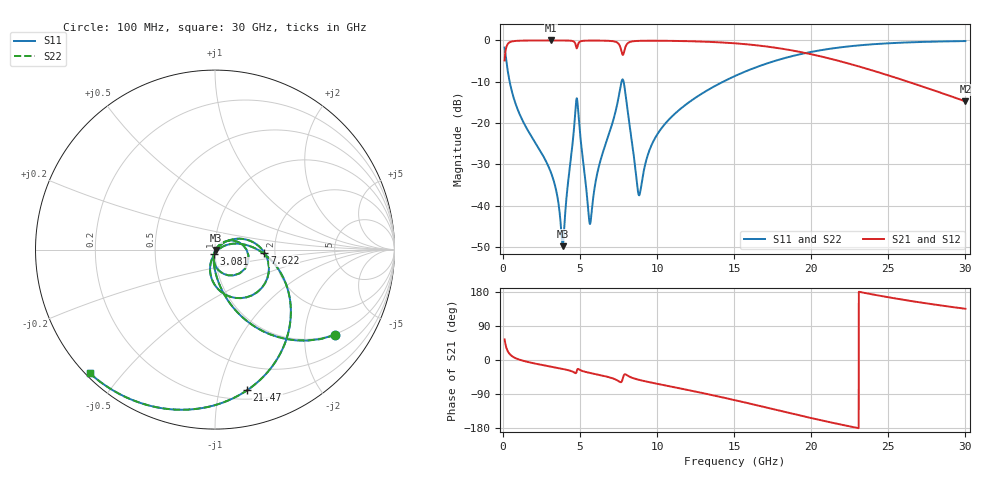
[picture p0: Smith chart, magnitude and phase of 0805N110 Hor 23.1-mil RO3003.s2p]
# GHz S MA R 50
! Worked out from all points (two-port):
!   3201 points, 100 MHz to 30 GHz, reference 50 ohm
!   highest |S21| = -0.02 dB at 3.09 GHz (marker M1); lowest = -14.8 dB at 30 GHz (marker M2)
!   |S21| within 3 dB of the highest: 143.3 MHz to 7.71 GHz (7.567 GHz wide, 193 % of centre); 7.835 GHz to 19.57 GHz (11.73 GHz wide, 85.6 % of centre)
!   lowest |S11| = -49.8 dB at 3.875 GHz (marker M3), VSWR 1.01, Z = 50.3 - j0.137 ohm
!   |S11| at or under -10 dB: 427.9 MHz to 7.687 GHz (7.259 GHz wide, 179 % of centre); 7.822 GHz to 14.28 GHz (6.463 GHz wide, 58.5 % of centre)
!   |S22| runs from -49.8 to -0.2 dB; largest |S21 - S12| = 0
!   S11 on the Smith chart (normalised r, x): 100 MHz: 0.97, -2.83; 3.081 GHz: 0.99, -0.05; 7.622 GHz: 1.76, -0.07; 21.47 GHz: 0.27, -1.22; 30 GHz: 0.01, -0.41
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0.1  0.8201 -35.5  0.5717 54.5  0.5717 54.5  0.8201 -35.5
0.3429375  0.3847 -69.4  0.9224 20.5  0.9224 20.5  0.3847 -69.4
0.62325  0.2218 -80.8  0.9742 9.0  0.9742 9.0  0.2218 -80.8
3.080656  0.02584 -102.7  0.9975 -17.4  0.9975 -17.4  0.02584 -102.7
3.09  0.02557 -102.7  0.9975 -17.5  0.9975 -17.5  0.02557 -102.7
3.874875  0.003219 -25.0  0.9966 -23.7  0.9966 -23.7  0.003219 -25.0
4.725156  0.1676 4.4  0.8643 -34.8  0.8643 -34.8  0.1676 4.4
4.865312  0.1456 -69.5  0.8931 -23.6  0.8931 -23.6  0.1456 -69.5
5.089563  0.05042 -97.9  0.9812 -28.2  0.9812 -28.2  0.05042 -97.9
5.528719  0.008627 -74.7  0.9933 -33.2  0.9933 -33.2  0.008627 -74.7
5.668875  0.006206 -15.3  0.9939 -34.4  0.9939 -34.4  0.006206 -15.3
6.182781  0.028 39.3  0.9937 -38.9  0.9937 -38.9  0.028 39.3
7.621719  0.2763 -3.7  0.8148 -58.6  0.8148 -58.6  0.2763 -3.7
7.892688  0.2634 -75.5  0.7782 -37.8  0.7782 -37.8  0.2634 -75.5
8.817719  0.0133 -46.0  0.9865 -52.3  0.9865 -52.3  0.0133 -46.0
9.434406  0.04327 20.5  0.9902 -58.0  0.9902 -58.0  0.04327 20.5
10.06978  0.07584 21.2  0.9896 -63.4  0.9896 -63.4  0.07584 21.2
15.05  0.3703 -17.2  0.9209 -106.1  0.9209 -106.1  0.3703 -17.2
20.03956  0.7271 -64.3  0.6764 -153.6  0.6764 -153.6  0.7271 -64.3
21.46916  0.8038 -77.1  0.5844 -166.5  0.5844 -166.5  0.8038 -77.1
25.01978  0.9221 -105.1  0.3758 165.5  0.3758 165.5  0.9221 -105.1
30  0.9805 -135.4  0.1825 135.2  0.1825 135.2  0.9805 -135.4
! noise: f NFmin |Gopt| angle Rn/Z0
0.1  0.0006995  0.912  0.9671  0.001749
3.417  0.006827  0.724  20.95  0.004752
6.743  0.01801  0.7918  40.44  0.01574
10.06  0.01971  0.736  58.78  0.01141
13.39  0.02225  0.7077  75.27  0.009551
16.7  0.02809  0.7225  90.31  0.01024
20.03  0.03622  0.7509  104.3  0.01142
23.35  0.04767  0.7875  117.4  0.01296
26.67  0.06481  0.8294  130  0.01485
30  0.09222  0.8727  142.5  0.01679
